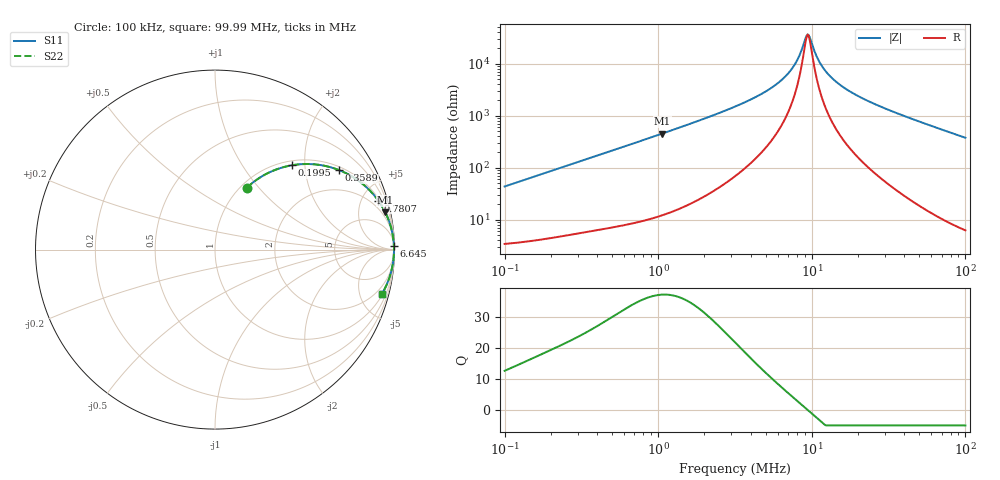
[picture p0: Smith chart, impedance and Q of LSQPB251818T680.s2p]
! LSQPB251818T680  S-PARAMETER MODEL  ( General Type )
! Model Generated by TAIYO YUDEN Corporation (http://www.ty-top.com)
! Version 2.0
! TAIYO YUDEN Control No. 100810NG19SB-FKC
! Copyright(c) 2009 TAIYO YUDEN CO.,LTD. All Rights Reserved.
! Product Description (link to TY-COMPAS)
! https://ds.yuden.co.jp/TYCOMPAS/or/detail?pn=LSQPB251818T680K&u=M
! Products Name : Inductors
! Characteristics :
!  Inductance : 68 uH , SRF(min) : 5.5 MHz , DC Resistance(max) : 3.12 Ohm
!  Rated Current : Saturation :340 mA , Temp Rise : 230 mA (40 degC)
!  Case Size : 2.5 x 1.8 / 0.098 x 0.071 [mm/inch] , Thickness : 1.8 / 0.071 [mm/inch]
!  (Conditions: Temperature = 25 degC , DC Bias Current/Voltage = 0A / 0V)
! External Node Assignments :
!  1  o---GGG---o  2
! GND o---------o GND
! Frequency Range : 0.1MHz  -  99.992428MHz  [ 402 STEP ]
# MHz S RI R 50
! Freq[MHz].  S11 Real  S11 Imag  S21 Real  S21 Imag  S12 Real  S12 Imag  S22 Real  S22 Imag
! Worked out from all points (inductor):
!   401 points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, 100 kHz to 99.99 MHz, reference 50 ohm
!   read as one part in series: L = 68.5 uH near 103.5 kHz
!   highest Q = 37.4 at 1.065 MHz (marker M1), where L = 67.7 uH
!   self-resonance near 9.386 MHz
!   S11 on the Smith chart (normalised r, x): 100 kHz: 1.07, +0.86; 199.5 kHz: 1.09, +1.71; 358.9 kHz: 1.12, +3.05; 780.7 kHz: 1.19, +6.61; 6.645 MHz: open; 99.99 MHz: 1.12, -7.50
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0.1  0.1765 0.3439  0.8235 -0.3439  0.8235 -0.3439  0.1765 0.3439
0.199525  0.4264 0.4695  0.5736 -0.4695  0.5736 -0.4695  0.4264 0.4695
0.318049  0.6415 0.4595  0.3585 -0.4595  0.3585 -0.4595  0.6415 0.4595
0.358917  0.6925 0.4425  0.3075 -0.4425  0.3075 -0.4425  0.6925 0.4425
0.524798  0.8237 0.3652  0.1763 -0.3652  0.1763 -0.3652  0.8237 0.3652
0.780711  0.9098 0.2728  0.0902 -0.2728  0.0902 -0.2728  0.9098 0.2728
1.011554  0.9434 0.2181  0.0566 -0.2181  0.0566 -0.2181  0.9434 0.2181
1.065341  0.9485 0.2081  0.0515 -0.2081  0.0515 -0.2081  0.9485 0.2081
3.162158  0.9925 0.0662  0.00747 -0.0662  0.00747 -0.0662  0.9925 0.0662
4.95429  0.996 0.0346  0.00403 -0.0346  0.00403 -0.0346  0.996 0.0346
6.644771  0.9969 0.0179  0.00309 -0.0179  0.00309 -0.0179  0.9969 0.0179
7.89731  0.9972 0.00894  0.00282 -0.00894  0.00282 -0.00894  0.9972 0.00894
9.225257  0.9973 0.00106  0.00273 -0.00106  0.00273 -0.00106  0.9973 0.00106
9.549449  0.9973 -0.000679  0.00273 0.000679  0.00273 0.000679  0.9973 -0.000679
10.05722  0.9973 -0.00329  0.00273 0.00329  0.00273 0.00329  0.9973 -0.00329
10.7765  0.9972 -0.00679  0.00277 0.00679  0.00277 0.00679  0.9972 -0.00679
11.54722  0.9972 -0.0103  0.00283 0.0103  0.00283 0.0103  0.9972 -0.0103
12.58859  0.9971 -0.0148  0.00294 0.0148  0.00294 0.0148  0.9971 -0.0148
14.20615  0.9968 -0.0213  0.00318 0.0213  0.00318 0.0213  0.9968 -0.0213
19.72309  0.9956 -0.0406  0.0044 0.0406  0.0044 0.0406  0.9956 -0.0406
31.98693  0.9911 -0.0776  0.00893 0.0776  0.00893 0.0776  0.9911 -0.0776
99.99243  0.9301 -0.2468  0.0699 0.2468  0.0699 0.2468  0.9301 -0.2468
